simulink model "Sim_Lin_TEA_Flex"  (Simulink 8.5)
settings: Solver=ode23  StartTime=0.0  StopTime=25*3600  RelTol=1e-3
InitFcn:
  | start
StopFcn:
  | pl2
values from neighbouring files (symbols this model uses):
  Kpqr = lqr(sys,Q0,R0)    [des.m]
  wo = 0.0011    [start.m]    (also in start1.m; start2.m; start3.m)
undefined symbols (not defined in the file or in its folder): Af, Bf, Cf, Df

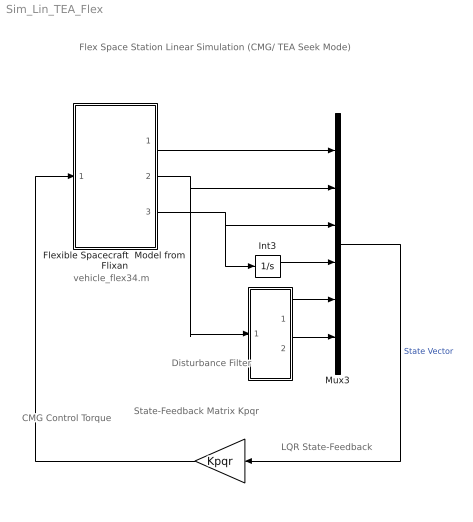
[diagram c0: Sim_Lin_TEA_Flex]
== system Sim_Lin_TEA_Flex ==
  note: LQR State-Feedback
  note: Flex Space Station Linear Simulation (CMG/ TEA Seek Mode)
  note: State-Feedback Matrix Kpqr
  note: CMG Control Torque
  note: Disturbance Filter
  note: vehicle_flex34.m
  " " : Gain  Gain=Kpqr  Multiplication=Matrix(K*u)
  "  " : Subsystem
  Flexible Spacecraft  Model from Flixan : Subsystem
  Int3 : Integrator
  Mux3 : Mux  Inputs=[3, 3, 3, 3, 1, 1]
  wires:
  Int3/1 -> Mux3/4
  " "/1 -> Flexible Spacecraft  Model from Flixan/1(Tcmg)
  Mux3/1 -> " "/1  "State Vector"
  "  "/1(a1) -> Mux3/5
  "  "/2(a2) -> Mux3/6
  Flexible Spacecraft  Model from Flixan/3("Hcmg ") -> Int3/1, Mux3/3
  Flexible Spacecraft  Model from Flixan/2(att-lv) -> "  "/1(the), Mux3/2
  Flexible Spacecraft  Model from Flixan/1(w-lv) -> Mux3/1

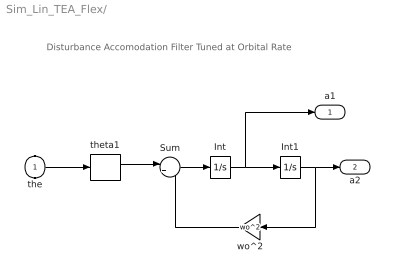
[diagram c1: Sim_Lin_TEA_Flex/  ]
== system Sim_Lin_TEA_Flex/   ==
  note: Disturbance Accomodation Filter Tuned at Orbital Rate
  the : Inport
  Int : Integrator
  Int1 : Integrator
  Sum : Sum  Inputs=|+-
  theta1 : Selector  InputPortWidth=3  Indices=[2]
  wo^2 : Gain  Gain=wo^2
  a1 : Outport
  a2 : Outport  Port=2
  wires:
  Int/1 -> Int1/1, a1/1
  Sum/1 -> Int/1
  Int1/1 -> wo^2/1, a2/1
  wo^2/1 -> Sum/2
  theta1/1 -> Sum/1
  the/1 -> theta1/1

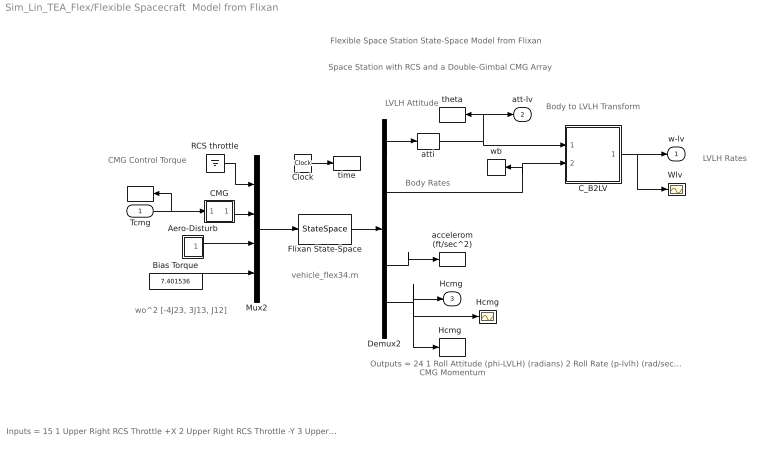
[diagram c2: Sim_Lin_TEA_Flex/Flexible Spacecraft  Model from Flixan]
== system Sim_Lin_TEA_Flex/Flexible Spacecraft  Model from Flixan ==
  note: Flexible Space Station State-Space Model from Flixan
  note: Space Station with RCS and a Double-Gimbal CMG Array
  note: wo^2 [-4J23, 3J13, J12]
  note: Inputs = 15 1 Upper Right RCS Throttle +X 2 Upper Right RCS Throttle -Y 3 Upper Left RCS Throttle +X 4 Upper Left RCS Throttle +Y 5 Lower Right RCS Throttle +X 6 Lower Right RCS Throttle -Y 7 Lower Left RCS Throttle +X 8 Lower Left RCS Throttle +Y 9 Double Gimbal CMG Torque in the X-axis (ft-lb) 10 Double Gimbal CMG Torque in the Y-axis (ft-lb) 11 Double Gimbal CMG Torque in the Z-axis (ft-lb) 12 External Torque Input 1 (ft-lb), direct: 13 External Torque Input 2 (ft-lb), direct: 14 External Torque Input 3 (ft-lb), direct: 15 Ext Torque Direct.=(0.197, -0.5964, -0.7782)
  note: CMG Momentum
  note: LVLH Attitude
  note: LVLH Rates
  note: Body to LVLH Transform
  note: Body Rates
  note: CMG Control Torque
  note: vehicle_flex34.m
  note: Outputs = 24 1 Roll Attitude (phi-LVLH) (radians) 2 Roll Rate (p-lvlh) (rad/sec) 3 Pitch Attitude (thet-LVLH) (radians) 4 Pitch Rate (q-lvlh) (rad/sec) 5 Yaw Attitude (psi-LVLH) (radians) 6 Yaw Rate (r-lvlh) (rad/sec) 7 Angle of attack, alfa, (radians) 8 Angle of sideslip, beta, (radian) 9 Change in Altitude, delta-h, (feet) 10 Forward Acceleration (V-dot) (ft/sec) 11 Cross Range Velocity (Vcr) (ft/sec) 12 Rate-Gyro # 1, Roll Rate (Body) (rad/sec) 13 Rate-Gyro # 2, Pitch Rate (Body) (rad/sec) 14 Rate-Gyro # 3, Yaw Rate (Body) (rad/sec) 15 Gyro # 4, Roll Attitude (Body) (radians) 16 Gyro # 5, Pitch Attitude (Body) (radians) 17 Gyro # 6, Yaw Attitude (Body) (radians) 18 Accelerom # 1, (along X), (ft/sec^2) Translat. Accelerat. 19 Accelerom # 2, (along Z), (ft/sec^2) Translat. Accelerat. 20 Accelerom # 3, (along X), (ft/sec^2) Translat. Accelerat. 21 Accelerom # 4, (along Z), (ft/sec^2) Translat. Accelerat. 22 Double Gimbal CMG Momentum Change in X-axis (ft-lb-sec) 23 Double Gimbal CMG Momentum Change in Y-axis (ft-lb-sec) 24 Double Gimbal CMG Momentum Change in Z-axis (ft-lb-sec)
  Tcmg : Inport  PortDimensions=3
  "   " : ToWorkspace  VariableName=Tcmg  SampleTime=-1
  Aero-Disturb : Subsystem
  Bias Torque : Constant  Value=7.401536
  CMG : Subsystem
  C_B2LV : Subsystem
  Clock : Clock
  Demux2 : Demux  Outputs=[11, 3, 3, 4, 3]
  Flixan State-Space : StateSpace  A=Af  B=Bf  C=Cf  D=Df  X0=0
  Hcmg : Scope
  "Hcmg  " : ToWorkspace  VariableName=Hcmg  SampleTime=-1
  Mux2 : Mux  Inputs=[8, 3, 3, 1]
  RCS throttle : Ground
  "Wlv " : Scope
  accelerom (ft/sec^2) : ToWorkspace  VariableName=accel  SampleTime=-1
  atti : Selector  InputPortWidth=11  Indices=[1 3 5]
  theta : ToWorkspace  VariableName=theta  SampleTime=-1
  time : ToWorkspace  VariableName=time  SampleTime=-1
  wb : ToWorkspace  VariableName=wb  SampleTime=-1
  w-lv : Outport
  att-lv : Outport  Port=2
  "Hcmg " : Outport  Port=3
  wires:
  Mux2/1 -> Flixan State-Space/1
  Flixan State-Space/1 -> Demux2/1
  Bias Torque/1 -> Mux2/4
  Clock/1 -> time/1
  RCS throttle/1 -> Mux2/1
  Demux2/5 -> "Hcmg "/1, Hcmg/1, "Hcmg  "/1
  Demux2/1 -> atti/1
  Demux2/4 -> accelerom (ft/sec^2)/1
  Tcmg/1 -> CMG/1(I), "   "/1
  Aero-Disturb/1(Td) -> Mux2/3
  CMG/1(O) -> Mux2/2
  atti/1 -> theta/1, att-lv/1, C_B2LV/1(atti)
  Demux2/2 -> C_B2LV/2(wb), wb/1
  C_B2LV/1(wlv) -> "Wlv "/1, w-lv/1

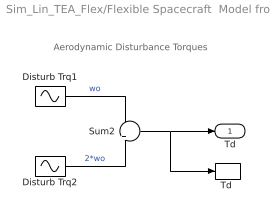
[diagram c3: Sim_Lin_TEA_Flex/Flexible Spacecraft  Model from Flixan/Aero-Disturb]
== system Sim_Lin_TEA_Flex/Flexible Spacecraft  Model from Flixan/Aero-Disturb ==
  note: Aerodynamic Disturbance Torques
  Disturb Trq1 : Sin  Amplitude=[1, 3, 1]  Bias="[1  8  1]"  Frequency=[wo, wo, wo]  SampleTime=0
  Disturb Trq2 : Sin  Amplitude=[1, 1, 1]*0.5  Frequency=[wo, wo, wo]*2  SampleTime=0
  Sum2 : Sum  Inputs=+|+
  "Td " : ToWorkspace  VariableName=Td  SampleTime=-1
  Td : Outport
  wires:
  Disturb Trq1/1 -> Sum2/1  "wo"
  Sum2/1 -> Td/1, "Td "/1
  Disturb Trq2/1 -> Sum2/2  "2*wo"

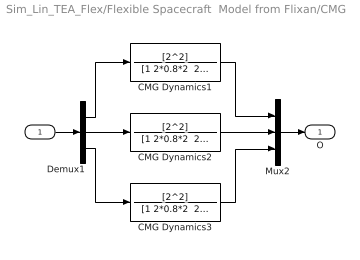
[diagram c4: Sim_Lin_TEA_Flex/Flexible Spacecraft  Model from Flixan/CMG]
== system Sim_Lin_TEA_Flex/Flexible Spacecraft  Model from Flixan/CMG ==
  I : Inport
  CMG Dynamics1 : TransferFcn  Numerator=[2^2]  Denominator="[1 2*0.8*2  2^2]"
  CMG Dynamics2 : TransferFcn  Numerator=[2^2]  Denominator="[1 2*0.8*2  2^2]"
  CMG Dynamics3 : TransferFcn  Numerator=[2^2]  Denominator="[1 2*0.8*2  2^2]"
  Demux1 : Demux  Outputs=3
  Mux2 : Mux  Inputs=3
  O : Outport
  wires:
  Mux2/1 -> O/1
  I/1 -> Demux1/1
  Demux1/3 -> CMG Dynamics3/1
  Demux1/1 -> CMG Dynamics1/1
  Demux1/2 -> CMG Dynamics2/1
  CMG Dynamics1/1 -> Mux2/1
  CMG Dynamics3/1 -> Mux2/3
  CMG Dynamics2/1 -> Mux2/2

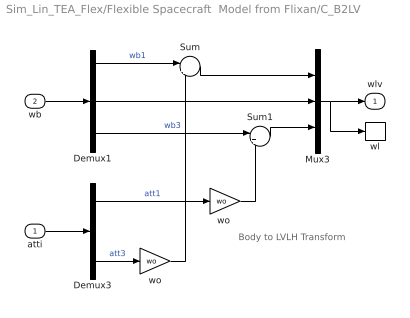
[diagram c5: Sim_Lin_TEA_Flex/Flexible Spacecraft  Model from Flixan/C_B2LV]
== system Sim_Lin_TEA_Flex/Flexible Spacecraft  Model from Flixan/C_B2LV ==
  note: Body to LVLH Transform
  atti : Inport  PortDimensions=3
  wb : Inport  Port=2  PortDimensions=3
  Demux1 : Demux  Outputs=3
  Demux3 : Demux  Outputs=3
  Mux3 : Mux  Inputs=3
  Sum : Sum  Inputs=|++
  Sum1 : Sum  Inputs=|+-
  wl : ToWorkspace  VariableName=wl  SampleTime=-1
  wo : Gain  Gain=wo
  "wo " : Gain  Gain=wo
  wlv : Outport
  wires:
  "wo "/1 -> Sum1/2
  Demux1/3 -> Sum1/1  "wb3"
  wo/1 -> Sum/2
  Demux1/2 -> Mux3/2
  Demux3/1 -> "wo "/1  "att1"
  Mux3/1 -> wl/1, wlv/1
  wb/1 -> Demux1/1
  atti/1 -> Demux3/1
  Sum1/1 -> Mux3/3
  Demux3/3 -> wo/1  "att3"
  Sum/1 -> Mux3/1
  Demux1/1 -> Sum/1  "wb1"
